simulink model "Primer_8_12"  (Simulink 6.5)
settings: Solver=ode23t  StartTime=0.0  StopTime=0.1  RelTol=1e-4
undefined symbols (not defined in the file or in its folder): blocks, Continuous, powergui, ZData
libraries: powerlib x6

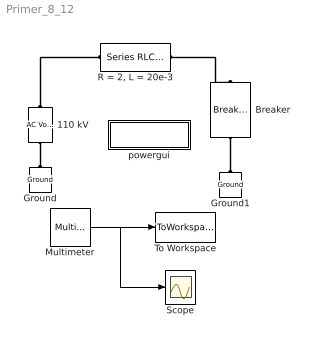
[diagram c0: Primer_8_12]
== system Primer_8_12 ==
  110 kV : powerlib/Electrical Sources/AC Voltage Source  Orientation=up  DialogController=PMDialogs.PMDefaultMaskDlg  SystemSampleTime=-1  Amplitude=110e3/sqrt(3)*sqrt(2)  Phase=0  Frequency=50  SampleTime=0  Measurements=None
  Breaker : powerlib/Elements/Breaker  Orientation=up  DialogController=PMDialogs.PMDefaultMaskDlg  SystemSampleTime=-1  BreakerResistance=0.01  InitialState=0  SnubberResistance=1e6  SnubberCapacitance=inf  SwitchingTimes=Tvkl  External=off  Measurements=None  MoreParameters=off  NoBreakLoop=off
  Ground : powerlib/Elements/Ground  Orientation=down  DialogController=PMDialogs.PMDefaultMaskDlg  PhysicalDomain=powersysdomain  SubClassName=unknown  LeftPortType=p1  RightPortType=p1  LConnTagsString=a
  Ground1 : powerlib/Elements/Ground  Orientation=down  DialogController=PMDialogs.PMDefaultMaskDlg  PhysicalDomain=powersysdomain  SubClassName=unknown  LeftPortType=p1  RightPortType=p1  LConnTagsString=a
  Multimeter : powerlib/Measurements/Multimeter  SystemSampleTime=-1  PhasorSimulation=off  OutputType=Complex  sel=1  L=1  Gain=1  yselected={'Ib: R = 2, L = 20e-3'};  PSBOutputType=1  PSBequivalent=0  AxesSetting=[0,0.1,-100,100]  Display=0  SavedBlockNames=-11
  "R = 2, L = 20e-3" : powerlib/Elements/Series RLC Branch  DialogController=PMDialogs.PMDefaultMaskDlg  PhysicalDomain=powersysdomain  SubClassName=unknown  LeftPortType=p1  RightPortType=p1  LConnTagsString=__new0  RConnTagsString=__new0  BranchType=RL  Resistance=2  Inductance=20e-3  SetiL0=on  InitialCurrent=0  Capacitance=1e-6  Setx0=off  InitialVoltage=0  Measurements=Branch current
  Scope : Scope
  To Workspace : ToWorkspace  VariableName=struja  SampleTime=-1  SaveFormat=Array
  powergui : Subsystem  AncestorBlock=powerlib/powergui  InitFcn=powergui( 'InitFcn_Callback' , gcb , 0 , [ ] );  mask(PSB option menu block){SimulationMode=Continuous, SampleTime=50e-6, echomessages=off, RestoreLinks=warning, x0status=blocks, Frange=[0:2:500], Ylog=off, Xlog=on, ShowGrid=off, save=off, variable=ZData, structure=, ZoomFFT=on, StartTime=0.0, cycles=1, DisplayStyle=1, fundamental=60, FreqAxis=off, MaxFrequency=1000, frequencyindice=50, frequencyindicesteady=1, RmsSteady=1, display=off, Ts=0, frequency=60, methode=off, HookPort=off, Interpol=off}
      mask prompts: SimulationMode "Simulation mode"; SampleTime "Sample time Ts (when simulation mode is Discrete) (s)"; echomessages "Echo  Messages"; RestoreLinks "Restore disabled links"; x0status "Initial electrical states status"; Frange "Impedance tool: Frequency Range"; Ylog "Impedance tool: Log impedance"; Xlog "Impedance tool: log Frequency"; ShowGrid "Impedance tool: grid"; save "Impedance tool: Save Data To Workspace"; variable "Impedance tool: Variable Name"; structure "Structure Name (PSBFFTSCOPE)"; ZoomFFT "ZoomFFT (PSBFFTSCOPE)"; StartTime "Start Time (PSBFFTSCOPE)"; cycles "Cycles (PSBFFTSCOPE)"; DisplayStyle "Display style (PSBFFTSCOPE)"; fundamental "Fundamental (PSBFFTSCOPE)"; FreqAxis "Frequency Axis (PSBFFTSCOPE)"; MaxFrequency "Max Frequency (PSBFFTSCOPE)"; frequencyindice "Load flow frequency (Hz)"; frequencyindicesteady "Frequency indice (STEADYSTATE)"; RmsSteady "RMS display (STEADYSTATE)"; display "Display Results"; Ts "OBSOLETE 1"; frequency "Phasor frequency (Hz)"; methode "Phasor simulation"; HookPort "Hook port"; Interpol "Interpolate"
      mask init:
      | powerlibroot = which('powersysdomain');
      | PSBroot = powerlibroot(1:end-16);
      | %
      | switch SimulationMode
      | 	case 1
      | 		message=sprintf('Continuous');
      | 	case 2
      |         SampleTimeeval=evalin('base',SampleTime,'NaN');
      |         if isnan(SampleTimeeval)
      |             message=sprintf('Warning !!,\nUndefined sample time');
      |         else
      |             message=sprintf('Discrete,\nTs = %.4g s.',SampleTimeeval);
      |         end
      | 	case 3
      | 		message=sprintf('Phasors');
      | end
      | if strcmp(bdroot,'powerlib')
      |   message='powergui';
      | end
      | power_initmask();
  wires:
  Multimeter/1 -> To Workspace/1, Scope/1
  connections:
  110 kV/RConn1 -- "R = 2, L = 20e-3"/LConn1
  Ground1/LConn1 -- Breaker/LConn1
  Ground/LConn1 -- 110 kV/LConn1
  "R = 2, L = 20e-3"/RConn1 -- Breaker/RConn1

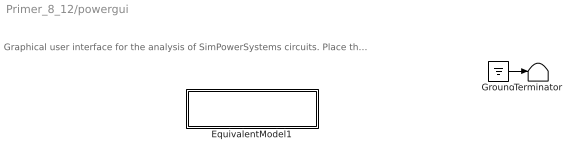
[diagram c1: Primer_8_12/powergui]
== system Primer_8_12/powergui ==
  note: Graphical user interface for the analysis of SimPowerSystems circuits. Place the Powergui block in the top-level of your model and double-click on it to open the GUI.
  EquivalentModel1 : Subsystem
  Ground : Ground
  Terminator : Terminator
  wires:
  Ground/1 -> Terminator/1

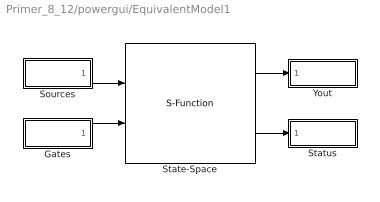
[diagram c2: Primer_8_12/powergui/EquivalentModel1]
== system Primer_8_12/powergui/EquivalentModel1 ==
  Gates : Subsystem
  Sources : Subsystem
  State-Space : S-Function  FunctionName=sfun_spssw_contc  Parameters=A, B, C, D, x0, SwitchResistance ,SwitchType, SwitchGateInitialValue, OutputsToResetToZero
  Status : Subsystem
  Yout : Subsystem
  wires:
  Gates/1(gates) -> State-Space/2
  Sources/1(u) -> State-Space/1
  State-Space/2 -> Status/1(status)
  State-Space/1 -> Yout/1(v,i)

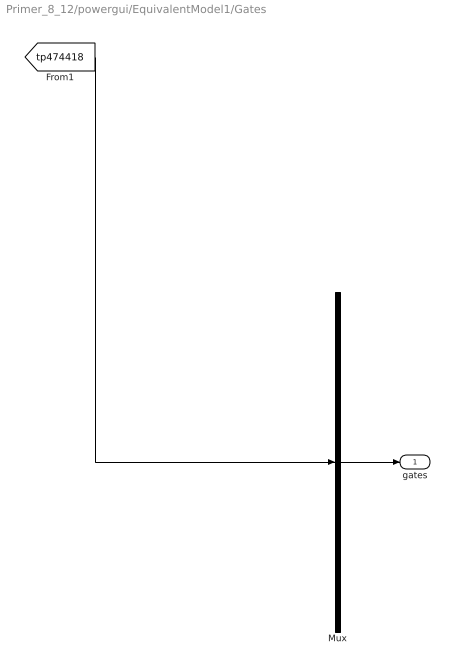
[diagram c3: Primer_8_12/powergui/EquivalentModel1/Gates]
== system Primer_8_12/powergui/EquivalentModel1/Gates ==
  Mux : Mux  Inputs=1
  gates : Outport
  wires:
  Mux/1 -> gates/1
  [tp474418] -> Mux/1

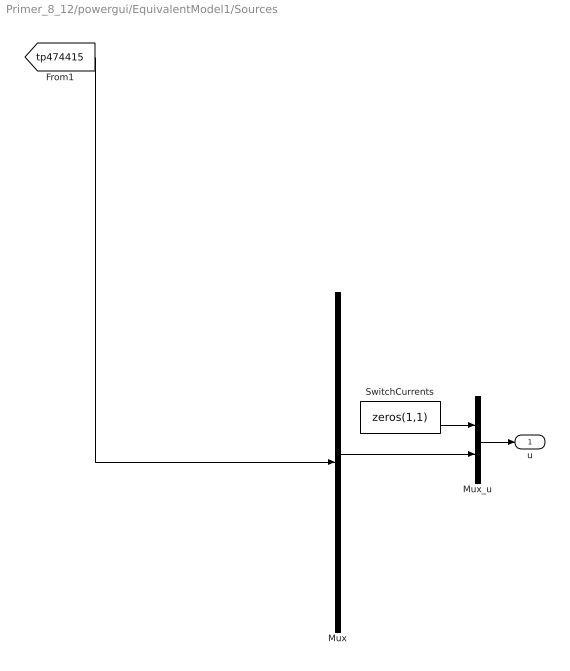
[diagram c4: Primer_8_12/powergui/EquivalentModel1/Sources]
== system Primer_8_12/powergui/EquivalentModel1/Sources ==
  Mux : Mux  Inputs=1
  Mux_u : Mux  Inputs=[1 1]
  SwitchCurrents : Constant  Value=zeros(1,1)  OutDataType=sfix(16)  ConRadixGroup=Use specified scaling  OutScaling=2^0  SampleTime=inf  FramePeriod=inf
  u : Outport
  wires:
  Mux/1 -> Mux_u/2
  SwitchCurrents/1 -> Mux_u/1
  Mux_u/1 -> u/1
  [tp474415] -> Mux/1

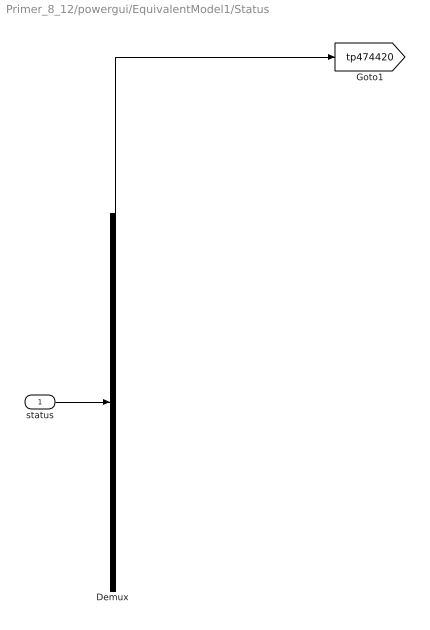
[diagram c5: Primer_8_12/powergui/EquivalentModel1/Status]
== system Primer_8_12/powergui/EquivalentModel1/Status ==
  status : Inport
  Demux : Demux  Outputs=1
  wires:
  status/1 -> Demux/1
  Demux/1 -> [tp474420]

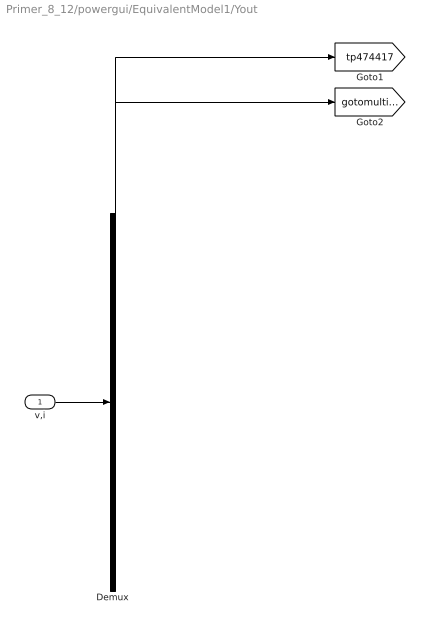
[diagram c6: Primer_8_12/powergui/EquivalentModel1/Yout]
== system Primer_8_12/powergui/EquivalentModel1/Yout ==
  v,i : Inport
  Demux : Demux  Outputs=[1 1]
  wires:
  v,i/1 -> Demux/1
  Demux/1 -> [tp474417]
  Demux/2 -> [gotomultimeterPSB]
